(* Logix 5000 Rung export; software revision 16.04 *)

MODULES
   Local : vendor None type None code None
   MVI56E_AFC : vendor None type None code None
END_MODULES

TYPE AFCEComponents :   // High precision gas component analysis (only supported version 2.07.000)
STRUCT
   C1 : REAL;   // Methane
   N2 : REAL;   // Nitrogen
   CO2 : REAL;   // Carbon Dioxide
   C2 : REAL;   // Ethane
   C3 : REAL;   // Propane
   H20 : REAL;   // Water
   H2S : REAL;   // Hydrogen Sulphide
   H2 : REAL;   // Hydrogen
   CO : REAL;   // Carbon Monoxide
   O2 : REAL;   // Oxygen
   IC4 : REAL;   // Iso-butane
   NC4 : REAL;   // Normal Butane
   IC5 : REAL;   // Iso-pentane
   NC5 : REAL;   // Normal-pentane
   C6 : REAL;   // Hexane
   C7 : REAL;   // Heptane
   C8 : REAL;   // Octane
   C9 : REAL;   // Nonane
   C10 : REAL;   // Decane
   He : REAL;   // Helium
   Ar : REAL;   // Argon
   NeoC5 : REAL;   // Not Used
   UxUser1 : REAL;   // Not Used
   UyUser2 : REAL;   // Not Used
   UxUser3 : REAL;   // Not Used
   UyUser4 : REAL;   // Not Used
   UxUser5 : REAL;   // Not Used
   UyUser6 : REAL;   // Not Used
   UxUser7 : REAL;   // Not Used
   UyUser8 : REAL;   // Not Used
   UxUser9 : REAL;   // Not Used
   UyUser10 : REAL;   // Not Used
END_STRUCT
END_TYPE

TYPE AFCEProveProcess :   // Prove process output from processor to the module
STRUCT
   Sequencing : AFCEProveSequencing;   // Prover sequencing
   Temperature : REAL;   // Temperature for Single Probe provers. And Inlet Temperature for Dual Probe Provers.
   OutletTemperature : REAL;   // Outlet Temperature for Provers with Dual Probes.
   SwitchBarTemperature : REAL;   // Switch bar temperature
   Pressure : REAL;   // Pressure for Single Probe provers. And Inlet Pressure for Dual Probe Provers.
   OutletPressure : REAL;   // Outlet Pressure for Provers with Dual Probes.
   ProverDensity : REAL;   // Prover density
END_STRUCT
END_TYPE

TYPE AFCEMeterControl :   // Enable/Disable Meter and Streams
STRUCT
   Meter : AFCEMeterControlMeter;   // Control the Meter
   Stream : AFCEMeterControlStream;   // Control the Meter Streams
   ResetAccumulators : AFCEMeterSignals;   // Resets for meter accumulators
END_STRUCT
END_TYPE

TYPE AFCEMeterDifferentialGasBackPlaneReturn :   // Differential Gas Meter
STRUCT
   StandardDefault : AFCEMeterDifferentialGasStandardDflt;
   StandardRaw : INT[14];
   Extended : AFCEExtended;
END_STRUCT
END_TYPE

TYPE AFCEModbusMasterDataType :   // Modbus master data type
STRUCT
   Bit : BOOL;   // bit type
   Word : BOOL;   // word type (16-bit)
   Long : BOOL;   // long integer (32-bit)
   LongRemote : BOOL;   // long integer (32-bit)
END_STRUCT
END_TYPE

TYPE AFCEProveSequencing :   // AFC prove sequencing tag for phase selection and ball positioning
STRUCT
   Phase : AFCEProvePhaseBitmap;   // AFC phase sequencing
   BallPositionReady : BOOL;   // Ball position: Ready (Udir & Bdir only; fwd leg Bdir)
   BallPositionSealed : BOOL;   // Ball position: Sealed (Udir & Bdir only; fwd leg Bdir)
   BallPositionReadyBwdLeg : BOOL;   // Ball position: Ready bwd leg (Bdir only)
   BallPositionSealedBwdLeg : BOOL;   // Ball position: Sealed bwd leg (Bdir only)
END_STRUCT
END_TYPE

TYPE AFCEUtil :   // Used for internal ladder logic usage. These values must not be changed by user application.
STRUCT
   Flags : AFCEFlag;   // Wallclock update commands
   CycleCounter : INT;   // Reflects current block ID calculated by ladder to be sent to the module
   Buffer : AFCEUtilBuffer;
   Block : AFCEUtilBlock;
END_STRUCT
END_TYPE

TYPE AFCEExtended :
STRUCT
   Trigger : BOOL;
   Data : AFCEExtendedData;
END_STRUCT
END_TYPE

TYPE AFCEModbusGatewayCommand :   // Modbus Gateway Command
STRUCT
   Config : AFCEModbusGatewayConfig;   // Config data to be entered by the user.
   Trigger : BOOL;   // Trigger the Command, when cleared module has responded.
   Data : INT[200];   // Contains modbus data written to the module (write commands)
END_STRUCT
END_TYPE

TYPE AFCEMeterDifferentialGasAlarmControl :   // Differential Gas Process Alarm Control
STRUCT
   DifferentialPressure : AFCEMeterProcessAlarm;   // Differential Pressure Alarms
   FlowRate : AFCEMeterProcessAlarm;   // Flow Rate Alarms
   Temperature : AFCEMeterProcessAlarm;   // Temperature Alarms
   Pressure : AFCEMeterProcessAlarm;   // Pressure Alarms
END_STRUCT
END_TYPE

TYPE AFCEMeterStatusStream :
STRUCT
   Active : INT;   // Current Active Stream
   Enabled : AFCEMeterStatusStreamEnabled;   // Enabled Streams
   Configured : AFCEMeterStatusStreamEnabled;   // Configured Streams
   EnableAlarm : AFCEMeterStatusStreamAlarm;   // Enable Alarms
END_STRUCT
END_TYPE

TYPE AFCEMeterDifferentialGasAlarm :   // Alarm Status and Control
STRUCT
   Control : AFCEMeterDifferentialGasAlarmControl;   // Alarm Control
END_STRUCT
END_TYPE

TYPE AFCEProveRunResults :   // Run results of the prove. Copied from the module to the pocessor
STRUCT
   CountAttempted : INT;   // Run count attempted
   CountCompleted : INT;   // Run count completed
   CountSelected : INT;   // Run count selected
   RunsSelected : INT;   // Bit Mapped Runs selected for calculations from completed runs
   NewMeterFactor : REAL;   // New meter factor
   ChangeInMeterFactor : REAL;   // Change in meter factor
END_STRUCT
END_TYPE

TYPE AFCEModbusMasterSwap :   // Modbus master swap words/ swap bytes
STRUCT
   SwapWords : BOOL;   // Swap words
   SwapBytes : BOOL;   // Swap bytes
END_STRUCT
END_TYPE

TYPE AFCEModbusMaster :   // Modbus Master. Port 3 must be configured as modbus master through AFC Manager to use this feature.
STRUCT
   Enable : BOOL;   // Enable the modbus master funcionality
   CommandIndex : INT;   // Selects which command index will be executed
   Command : AFCEModbusMasterCommand[10];   // Each command contains a specific modbus request to be sent out of the port
END_STRUCT
END_TYPE

TYPE AFCEFlag :   // Flags contains status information updated by ladder and also trigger bits for clock update
STRUCT
   AFCStopped : BOOL;   // Indicates that the module has sent a new input block to be processed by ladder - UPDATED BY LADDER
   AFCInputSequenceNum : INT;   // Meter number (0 -15) associated to blocks 1-16. Used to update "Profile" (meter type and product group.) UPDATED BY LADDER
END_STRUCT
END_TYPE

TYPE AFCEModbusPassThruBitData :   // AFC Modbus Pass-thru Bit Data
STRUCT
   Data : BOOL[2016];   // Contains received data for bit commands
END_STRUCT
END_TYPE

TYPE AFCEUtilBlockInterrupt :
STRUCT
   Now : BOOL;
   ModbusGateway : DINT;
   EnableDisable : BOOL;
   Analysis : DINT;
END_STRUCT
END_TYPE

TYPE AFCEMeterDifferentialGasArchiveFetchT :   // Fetch Archive
STRUCT
   Trigger : BOOL;   // Trigger Archive Fetch
   Age : INT;   // Initial Archive. 0 = Current Archive
   Error : AFCEMeterArchiveFetchError;   // Archive Fetch Error
   Default : AFCEMeterDifferentialGasArchiveDflt;   // Default Archive
   Raw : INT[100];   // Raw Archive
END_STRUCT
END_TYPE

TYPE AFCEFirmwareVersion :
STRUCT
   Major : SINT;   // Major Version number
   Minor : SINT;   // Minor Version number
   Revision : INT;   // Revision
END_STRUCT
END_TYPE

TYPE AFCEModbusGateway :   // Modbus Gateway
STRUCT
   Command : AFCEModbusGatewayCommand[10];   // Modbus gateway commands - contains setup and modbus data
END_STRUCT
END_TYPE

TYPE AFCEMeterCalRequestActionType :
STRUCT
   ZeroShift : BOOL;   // Zero Shift
   SetZero : BOOL;   // Set Zero
   SetSpan : BOOL;   // Set Span
   SetMid1 : BOOL;   // Set Mid 1
   SetMid2 : BOOL;   // Set Mid 2
   SetMid3 : BOOL;   // Set Mid 3
END_STRUCT
END_TYPE

TYPE AFCEUtilBuffer :   // Buffer
STRUCT
   Input : INT[250];   // Input buffer contains the complete block to be copied from the module
   Output : INT[248];   // Output buffer contains data the complete block to be copied to the module
   Process : INT[240];
   ArchiveDay : INT[98];
   ArchiveHour : INT[98];
   Prove : INT[26];
   Analysis : INT[198];
   MeterEnableDisable : INT[4];
   StreamEnable : INT[48];
   StreamDisable : INT[48];
   StreamSelect : INT[32];
   MeterSignals : INT[32];
   Calibration : INT[36];
END_STRUCT
END_TYPE

TYPE AFCEUtilBlock :
STRUCT
   ProcessInput : INT;
   InterruptPending : AFCEUtilBlockInterrupt;
   InterruptComplete : AFCEUtilBlockInterrupt;
   NonInterruptPending : AFCEUtilBlockNonInterrupt;
   NonInterruptComplete : AFCEUtilBlockNonInterrupt;
END_STRUCT
END_TYPE

TYPE AFCEMeterDifferentialGasCalRequestProces :
STRUCT
   DifferentialPressure : BOOL;   // Differential Pressure
   Temperature : BOOL;   // Temperature
   Pressure : BOOL;   // Pressure
END_STRUCT
END_TYPE

TYPE AFCEMeterSignals :   // Meter trigger accumulator and archive resets
STRUCT
   ResetAccumulator1 : BOOL;   // Set to 1 to reset resettable accumulator 1
   ResetAccumulator2 : BOOL;   // Set to 1 to reset resettable accumulator 2
   ResetAccumulator3 : BOOL;   // Set to 1 to reset resettable accumulator 3
   ResetAccumulator4 : BOOL;   // Set to 1 to reset resettable accumulator 4
END_STRUCT
END_TYPE

TYPE AFCEProve :   // Prove
STRUCT
   Process : AFCEProveProcess;   // Process Variables
   Signals : AFCEProveSignals;   // AFC Prove Signals (triggers the proving update)
   Config : AFCEProveConfig;   // AFC Prove Control (configuration settings)
   PulseCounts : AFCEProvePulseCount;   // Pulse counts to be updated at the end of the run/pass
   ConfigInput : AFCEProveInputConfig;   // AFC prover input configuration
   Status : AFCEProveStatus;   // AFC prover status
   ErrorCode : INT;   // Prove error code
   ProveControlsEcho : INT;   // AFC module Echos the state of the Prove Controls
   RequestedMeterEcho : INT;   // AFC module Echos the Meter number requested
   RequestedCurvePointEcho : INT;   // AFC module Echos the requested Curve Point
   RunResults : AFCEProveRunResults;   // Prove and run results
   ProveEnabled : BOOL;   // ON if prove is enabled. This flag is coped from inputbuffer[247]
END_STRUCT
END_TYPE

TYPE AFCEMeterControlStream :
STRUCT
   Selected : SINT;   // Stream to Enable or Disable and/or make active.
   EnableSelected : BOOL;   // Enable the Selected Stream
   DisableSelected : BOOL;   // Disable the Selected Stream
   SetSelectedToActive : BOOL;   // Set Selected to Active Stream
END_STRUCT
END_TYPE

TYPE AFCEProveConfig :   // Controls (configuration settings) associated to the prover
STRUCT
   Enable : AFCEProveConfigEnable;   // Controls at enable
   Accept : AFCEProveConfigAccept;   // Controls at accept
END_STRUCT
END_TYPE

TYPE AFCEWallclock :
STRUCT
   GetAFCTime : BOOL;   // Get current AFC Time
   SetAFCTimeFromPLCTime : BOOL;   // Set AFC time from PLC time. Updates current AFC time
   EnableLocalDateTime : BOOL;   // Enable Local Date Time.
   AFCTime : AFCETime;   // Coordinated Universal Time. Updated by either getting or setting AFC time.
END_STRUCT
END_TYPE

TYPE AFCEMeterDifferentialGasStandardDflt :   // Differential Gas Meter Default Standard Data
STRUCT
   Meter_Alarms : DINT;   // Meter alarms
   NR_Acc_Net_Totalizer : DINT;   // Non-resettable accumulator, net, totalizer (m3)
   NR_Acc_Net_Residue : REAL;   // Non-resettable accumulator, net, residue (m3)
   FlowRate_Net : REAL;   // Flow rate, net (m3/h)
   FlowRate_Gross : REAL;   // Flow rate, gross (m3/h)
   Ifpv : REAL;   // AGA 8, Supercompressibility, Fpv
   Cprime : REAL;   // C-prime
END_STRUCT
END_TYPE

TYPE AFCEMeterCalRequestActionValue :
STRUCT
   ZeroShift : AFCEMeterCalRequestValue;   // Zero Shift
   SetZero : AFCEMeterCalRequestValue;   // Set Zero
   SetSpan : AFCEMeterCalRequestValue;   // Set Span
   SetMid1 : AFCEMeterCalRequestValue;   // Set Mid 1
   SetMid2 : AFCEMeterCalRequestValue;   // Set Mid 2
   SetMid3 : AFCEMeterCalRequestValue;   // Set Mid 3
END_STRUCT
END_TYPE

TYPE AFCEMeterStatus :   // Status
STRUCT
   Meter : AFCEMeterStatusMeter;   // Meter Status
   Stream : AFCEMeterStatusStream;   // Stream Status
END_STRUCT
END_TYPE

TYPE AFCEModbusMasterConfig :   // Modbus master command settings
STRUCT
   Enable : BOOL;   // Set to 1 to enable command (0=disable)
   FunctionType : BOOL;   // Set to 1 to select write command (0=read command)
   RegisterBank : BOOL;   // Set to 1 to select input register (0=holding register)
   DataType : AFCEModbusMasterDataType;   // Select data type format
   SwapOption : AFCEModbusMasterSwap;   // Select byte and word swap (1 = swap, 0 = no swap)
   TypeSwap : INT;   // This value is calculated by ladder logic and must not be modified by user
   SlaveAddress : INT;   // Modbus slave address of remote device
   ModbusAddress : INT;   // Modbus data address on remote slave
   ElementCount : INT;   // Number of data elements (125 words)
   TransactionID : INT;   // Transaction ID. This value is returned to the ReturnedTransaction ID when the response has been received.
END_STRUCT
END_TYPE

TYPE AFCEMeterStatusStreamEnabled :   // Stream Status 1 = Enabled
STRUCT
   Stream1 : BOOL;
   Stream2 : BOOL;
   Stream3 : BOOL;
   Stream4 : BOOL;
   Stream5 : BOOL;
   Stream6 : BOOL;
   Stream7 : BOOL;
   Stream8 : BOOL;
   Stream9 : BOOL;
   Stream10 : BOOL;
   Stream11 : BOOL;
   Stream12 : BOOL;
   Stream13 : BOOL;
   Stream14 : BOOL;
   Stream15 : BOOL;
   Stream16 : BOOL;
END_STRUCT
END_TYPE

TYPE AFCEMeterDifferentialGasArchiveWrite :   // Write Archive
STRUCT
   Daily : BOOL;   // Set to 1 to write daily archive
   Hourly : BOOL;   // Set to 1 to write hourly archive
END_STRUCT
END_TYPE

TYPE AFCEMeterArchiveFetchError :
STRUCT
   ArchiveSelectionInvalid : BOOL;   // Archive File Selection Invalid
   AgeOutsideSize : BOOL;   // Age Outside Configured File Size
   ArchiveNeverWritten : BOOL;   // Age OK but Archive Record Never Written (new or reconfigured meter)
   Reserverd1 : BOOL;
   Reserverd2 : BOOL;
   Reserverd3 : BOOL;
   Reserverd4 : BOOL;
   Reserverd5 : BOOL;
   Reserverd6 : BOOL;
   Reserverd7 : BOOL;
   Reserverd8 : BOOL;
   Reserverd9 : BOOL;
   Reserverd10 : BOOL;
   Reserverd11 : BOOL;
   Reserverd12 : BOOL;
   Reserverd13 : BOOL;
END_STRUCT
END_TYPE

TYPE AFCEMeterDifferentialGasCalRequest :
STRUCT
   ProcessVariable : AFCEMeterDifferentialGasCalRequestProces;   // Process Variable
   ActionType : AFCEMeterCalRequestActionType;   // Action Type
   Value : AFCEMeterCalRequestActionValue;   // Value
   Count : DINT;   // Number of calibration requests
END_STRUCT
END_TYPE

TYPE AFCESiteStatus :   // Site status bits - contains general information about the module - not meter specific
STRUCT
   AFCActive : BOOL;   // AFC active
   ChecksumAlarms : BOOL;   // Checkum alarm active
   Reserved2 : BOOL;
   Reserved3 : BOOL;
   PLCHalted : BOOL;   // PLC in program mode or missing
   CfgChanged : BOOL;   // Configuration changed
   Powerup : BOOL;   // Module powered up
   ColdStart : BOOL;   // Module performed cold start (BBRAM initialized)
   ModbusMasterPending : BOOL;   // Modbus Master Poll Pending
   ModbusMasterComplete : BOOL;   // Modbus Master Poll Complete
   ModbusPassThruPending : BOOL;   // Modbus Pass-thru Input Pending
   CalibrationRequest : BOOL;   // Calibration request from module
   ProverEnabled : BOOL;   // Prover Enabled
   Reserved13 : BOOL;
   Reserved14 : BOOL;
   Reserved15 : BOOL;
END_STRUCT
END_TYPE

TYPE AFCEModuleDef :   // Main user defined data type
STRUCT
   ModbusGateway : AFCEModbusGateway;   // Reads and write data between processor and module modbus table
   ModbusMaster : AFCEModbusMaster;   // Setup modbus master commands to be sent to remote slaves (through Port 3)
   ModbusPassThru : AFCEModbusPassThru;   // Modbus pass-thru data
   SiteStatus : AFCESiteStatus;   // Site status
   MeterAlarms : AFCESiteAlarms;   // Meter Alarms
   Prove : AFCEProve;   // Prover
   Wallclock : AFCEWallclock;   // Set clock and get clock information
   Firmware : AFCEFirmwareVersion;   // Firmware information
   Util : AFCEUtil;   // Used by ladder logic
END_STRUCT
END_TYPE

TYPE AFCEModbusGatewayConfig :   // Modbus Ggateway Configuration
STRUCT
   Enable : BOOL;   // Set to 1 to enable modbus gateway command (0=disable)
   StartRegister : DINT;   // Start modbus address
   RegisterCount : INT;   // Word count (200 max)
   FunctionType : BOOL;   // 0 = read command, 1 = write command
   RegisterType : BOOL;   // 0 = holding register, 1 = input register
   SlaveType : BOOL;   // 0 = primary slave, 1 = virtual slave
END_STRUCT
END_TYPE

TYPE AFCEMeterCalRequestValue :
STRUCT
   Applied : REAL;   // Applied
   Measured : REAL;   // Measured
END_STRUCT
END_TYPE

TYPE AFCEUtilBlockNonInterrupt :
STRUCT
   Now : BOOL;
   ModbusMasterCommand : BOOL;
   ModbusMasterResponse : BOOL;
   Archive : DINT;
   Prover : BOOL;
   PassThru : BOOL;
   Calibration : BOOL;
END_STRUCT
END_TYPE

TYPE AFCEProveConfigAccept :   // Prove controls at accept. If auto-accept is selected must be available at enable
STRUCT
   RequestedInterpolationPoint : INT;   // Requested interpolation point (0 nearest)
   ApplyMFChangeAllStreams : BOOL;   // Apply change in meter factor to all streams
   ApplyMFChangeCurve : BOOL;   // Apply change in meter factor to all curve points
   ApplyNewMF : BOOL;   // CApply new meter factor
END_STRUCT
END_TYPE

TYPE AFCEMeterDifferentialGasProcess :   // Differential Gas Process Variables
STRUCT
   DifferentialPressure : REAL;   // Differential pressure if Primary Input = Differential pressure
   FlowRate : REAL;   // Flow Rate is Primary Input = Flow rate
   Temperature : REAL;   // Temperature
   Pressure : REAL;   // Static pressure
END_STRUCT
END_TYPE

TYPE AFCEProvePhaseBitmap :   // AFC prove phase bitmap
STRUCT
   NotSelected : BOOL;   // Not selected
   Active : BOOL;   // Active, not counting
   CountingPast1stSwitch : BOOL;   // Counting past 1st switch for Udir and forward leg for Bdir)
   Past2ndSwitchFwdLeg : BOOL;   // Past 2nd switch forward leg (bidirectional only)
   Past1stSwithRetLeg : BOOL;   // Past 1st switch return leg (bidirectional only)
   RunComplete : BOOL;   // Run complete. past 2nd switch.
END_STRUCT
END_TYPE

TYPE AFCETime :   // AFC time format used for wallclock update.
STRUCT
   Year : DINT;   // Year
   Month : DINT;   // Month
   Day : DINT;   // Day
   Hour : DINT;   // Hour
   Minute : DINT;   // Minute
   second : DINT;   // Seconds
END_STRUCT
END_TYPE

TYPE AFCEMeterDifferentialGasCal :   // Processor Mediated Calibration
STRUCT
   Request : AFCEMeterDifferentialGasCalRequest;   // Calibration Request from module
   Response : AFCEMeterCalResponse;   // Processor Response
END_STRUCT
END_TYPE

TYPE AFCEMeterDifferentialGasArchive :   // Different Gas Archive
STRUCT
   Write : AFCEMeterDifferentialGasArchiveWrite;
   Fetch : AFCEMeterDifferentialGasArchiveFetch;
END_STRUCT
END_TYPE

TYPE AFCEProveSignals :   // Contains the proving signals that will trigger specific tasks from the module
STRUCT
   EnableProve : BOOL;   // Enables the prove
   AcceptProve : BOOL;   // Accepts the prove
   RejectProve : BOOL;   // Reject the prove
   RunStart : BOOL;   // Starts the run
   RunComplete : BOOL;   // Flags that the run is complete
   RunCancel : BOOL;   // Cancels the run
   RunDelete : BOOL;   // Deletes the run
   PassComplete : BOOL;   // Flag that the pass is complete
   PauseProve : BOOL;   // Pauses the Proving Process
   AbortProve : BOOL;   // Aborts the prove
END_STRUCT
END_TYPE

TYPE AFCEMeterProfile :   // Meter configuration profile
STRUCT
   MeterType : BOOL;   // 0=Differential, 1=Linear
   ProductGroup : BOOL;   // 0=Gas, 1=Liquid
   PrimaryInput : BOOL;   // For differential, 0=Differential Pressure 1=Flow Rate. For Linear, 0=Pulse Count 1=Pulse Frequency
   AOIMismatch : BOOL;   // AOI Meter type does not match module for meter number
END_STRUCT
END_TYPE

TYPE AFCEMeterStatusStreamAlarm :   // Stream Alarms
STRUCT
   StreamOutOfRange : BOOL;   // Requested Stream Number Out of Range
   StreamNotConfigured : BOOL;   // Requested Stream not Configured
   StreamNotEnabled : BOOL;   // Requested Stream not Enabled
   EventLogFull : BOOL;   // Event Log Full, Action not Performed
END_STRUCT
END_TYPE

TYPE AFCEModbusPassThru :   // AFC Modbus Pass-thru
STRUCT
   Enable : BOOL;   // Set to 1 to enable pass-thru functionality (requires AFC Manager setting)
   MessagePresent : BOOL;   // Message present in the response block
   GetMessage : BOOL;   // Get the pass-thru message. When the bit is cleared the message has been transferred to the PLC.
   FunctionBitWrite : BOOL;   // Function bit write
   OverflowError : BOOL;   // Overflow error flag
   ModbusAddress : INT;   // Destination modbus address
   RegisterCount : INT;   // Number of elements associated to command
   ReadDataWord : INT[125];   // Contains received data for word commands
   ReadDataBit : AFCEModbusPassThruBitData;   // Contains received data for bit commands
END_STRUCT
END_TYPE

TYPE AFCEProveInputConfig :   // Prove input block results - prover configuration
STRUCT
   Type : INT;   // Prover type
   Options : INT;   // Prover options
   RunsPerProveTotal : INT;   // Total runs per prove
   RunsPerProveSelected : INT;   // Selected runs per prove
   MaxRunsBeforeAbort : INT;   // Max total runs before abort
   ShortPassesPerRun : INT;   // Short passes per run if bidir = 2 , else 0
END_STRUCT
END_TYPE

TYPE AFCEMeterDifferentialGasArchiveDflt :   // Default Configuration
STRUCT
   ClosingTimestamp : DINT;
   CumulativeActiveStreams : INT;
   CurrentActiveStream : SINT;
   MeterStatus : SINT;
   FlowingPeriod : DINT;
   PeriodDuration : DINT;
   AccumulatorTotalizer : DINT;
   AccumulatorResidue : REAL;
   MeterAlarms : DINT;
   PrimaryInput : REAL;   // Either Differential Pressure or Flow Rate
   Temperature : REAL;
   Pressure : REAL;
   RelativeDensity : REAL;
   ReferenceCompressibility : REAL;
   FlowingCompressibility : REAL;
   Fpv : REAL;
   PressureExtension : REAL;
   CoefficientDischarge : REAL;
   ExpansionFactor : REAL;
   Cprime : REAL;
   MassNRAccumulatorCurrent : REAL;   // Non-resettable
   MassNRAccumulatorOpening : REAL;   // Non-resettable
   EnergyNRAccumulatorCurrent : REAL;   // Non-resettable
   EnergyNRAccumulatorOpening : REAL;   // Non-resettable
   NetNRAccumulatorCurrent : REAL;   // Non-resettable
   NetNRAccumulatorOpening : REAL;   // Non-resettable
   GrossNRAccumulatorCurrent : REAL;   // Non-resettable
   GrossNRAccumulatorOpening : REAL;   // Non-resettable
   MolarFractionComponent01_C1 : REAL;
   MolarFractionComponent02_N2 : REAL;
   MolarFractionComponent03_CO2 : REAL;
   MolarFractionComponent04_C2 : REAL;
   MolarFractionComponent05_C3 : REAL;
   MolarFractionComponent06_H2O : REAL;
   MolarFractionComponent07_H2S : REAL;
   MolarFractionComponent08_H2 : REAL;
   MolarFractionComponent09_CO : REAL;
   MolarFractionComponent10_O2 : REAL;
   MolarFractionComponent11_IC4 : REAL;
   MolarFractionComponent12_NC4 : REAL;
   MolarFractionComponent13_IC5 : REAL;
   MolarFractionComponent14_NC5 : REAL;
   MolarFractionComponent15_C6 : REAL;
   MolarFractionComponent16_C7 : REAL;
   MolarFractionComponent17_C8 : REAL;
   MolarFractionComponent18_C9 : REAL;
   MolarFractionComponent19_C10 : REAL;
   MolarFractionComponent20_He : REAL;
   MolarFractionComponent21_Ar : REAL;
   UserSpecifiedFlowAveraged1 : REAL;
   UserSpecifiedFlowAveraged2 : REAL;
   UserSpecifiedFlowAveraged3 : REAL;
END_STRUCT
END_TYPE

TYPE AFCEProveStatus :   // Status of the prove (returned from the module to the processor)
STRUCT
   ProveAccepted : BOOL;   // Prove was accepted
   MeterFactorApplied : BOOL;   // Meter factor was applied
   MFAppliedToCurve : BOOL;   // Meter factor was applied to all points in the curve
   MFAppliedToStreams : BOOL;   // Meter factor was applied to all streams
   ProveRejectedByCommand : BOOL;   // Prove was rejected by command
   ProveRejectedNoRuns : BOOL;   // Prove was rejected - empty prove (no runs)
   ProveRejectedDivideBy0 : BOOL;   // Prove was rejected - divide by 0
   ProveEnabled : BOOL;   // Prove is enabled
   ProvingRunInProgress : BOOL;   // Proving run is in progress
   ProveRejectedAbort : BOOL;   // Prove rejected: abort
   ProvePaused : BOOL;   // Prove is paused
   RunCancelled : BOOL;   // Run Is cancelled
   RunTimedOut : BOOL;   // Run timed out
END_STRUCT
END_TYPE

TYPE AFCEMeterProcessAlarm :   // Process Alarms
STRUCT
   SetGeneralFail : BOOL;   // Set to indicate General Failure of the Transmitter
   StaleData : BOOL;   // Clear to Indicate new process input data
   SetLowThreshold : BOOL;   // Set to indicate Lower Range Limit Exceeded
   SetHighThreshold : BOOL;   // Set to indicate Upper Range Limit Exceeded
   SetAutoClearStaleData : BOOL;   // Set to automatically clear stale data
END_STRUCT
END_TYPE

TYPE AFCEProveConfigEnable :   // Prove controls at enable
STRUCT
   MeterNumber : INT;   // Meter number requested (1-16)
   AutoAcceptProve : BOOL;   // Auto-accept the prove
   AutoContinueProve : BOOL;   // Auto-continue the prove
END_STRUCT
END_TYPE

TYPE AFCEMeterAnalysis :   // Meter analysis components. Allows the processor to update molar analysis for low precision and high precision streams.
STRUCT
   Trigger : BOOL;   // Set to 1 to Send Updated Component Data to the Module
   Stream : INT;   // Stream for Analysis. Select 0 for current active stream.
   Error : AFCEMeterAnalysisError;   // Analysis Error
   Components : AFCEComponents;   // High precision gas components (floating point per component). Only supported for firmware version 2.07.000 or later
END_STRUCT
END_TYPE

TYPE AFCEMeterStatusMeter :   // Meter Status
STRUCT
   Enabled : BOOL;   // Meter Enable Status, 1=enabled
   EnableAlarm : BOOL;   // If set either: 1. The meter is not configured. 2. The event log is full, the action was not performed.
END_STRUCT
END_TYPE

TYPE AFCEMeterControlMeter :   // Enable and Disable Meter
STRUCT
   Enable : BOOL;   // Enable the Meter
   Disable : BOOL;   // Disable the Meter
END_STRUCT
END_TYPE

TYPE AFCEMeterDifferentialGas :   // Differential Gas Meter
STRUCT
   Control : AFCEMeterControl;   // Meter Control
   Status : AFCEMeterStatus;   // Meter Status
   ProcessVariables : AFCEMeterDifferentialGasProcess;   // Input process variables to be transferred to the module
   Analysis : AFCEMeterAnalysis;   // Molar Analysis data to be transferred to the module (only for gas products with online gas chromatograph applications)
   Alarm : AFCEMeterDifferentialGasAlarm;   // Meter Alarm status and control
   Archive : AFCEMeterDifferentialGasArchive;   // Archive
   Profile : AFCEMeterProfile;   // Module profile (meter type/product group) transfered from the module
   Calibration : AFCEMeterDifferentialGasCal;   // Calibration
   BackPlaneReturn : AFCEMeterDifferentialGasBackPlaneReturn;
END_STRUCT
END_TYPE

TYPE AFCEModbusMasterCommand :   // Modbus Master Command
STRUCT
   Config : AFCEModbusMasterConfig;   // Modbus Master Configuration
   ErrorCode : INT;   // Error Code associated to Modbus Master Command
   Pending : BOOL;   // Pending Modbus Master Command - waiting for Modbus Response
   ReturnedTransactionID : DINT;   // Changes to Config.TransactionID value when response has returned.
   Data : INT[100];   // Read or Write Data
END_STRUCT
END_TYPE

TYPE AFCEMeterDifferentialGasArchiveFetch :
STRUCT
   Daily : AFCEMeterDifferentialGasArchiveFetchT;
   Hourly : AFCEMeterDifferentialGasArchiveFetchT;
END_STRUCT
END_TYPE

TYPE AFCEProvePulseCount :   // Values to be supplied at the end of the pass/run
STRUCT
   Meter : DINT;   // Meter pulse count
   MasterMeter : DINT;   // Master meter pulse count
END_STRUCT
END_TYPE

TYPE AFCEMeterCalResponse :
STRUCT
   Trigger : BOOL;   // Send Error Code and Values to module to be recorded
   ErrorCode : SINT;   // Error Code to send. 0-4 allowed. 0=No error. 1-4=User defined.
   Value : AFCEMeterCalRequestValue;   // Value to Send
   Count : DINT;   // Number of calibration responses
END_STRUCT
END_TYPE

TYPE AFCEExtendedData :
STRUCT
   Raw : INT[64];
END_STRUCT
END_TYPE

TYPE AFCESiteAlarms :   // Indicates if a meter has any alarms
STRUCT
   Meter1 : BOOL;   // Meter in alarm
   Meter2 : BOOL;   // Meter in alarm
   Meter3 : BOOL;   // Meter in alarm
   Meter4 : BOOL;   // Meter in alarm
   Meter5 : BOOL;   // Meter in alarm
   Meter6 : BOOL;   // Meter in alarm
   Meter7 : BOOL;   // Meter in alarm
   Meter8 : BOOL;   // Meter in alarm
   Meter9 : BOOL;   // Meter in alarm
   Meter10 : BOOL;   // Meter in alarm
   Meter11 : BOOL;   // Meter in alarm
   Meter12 : BOOL;   // Meter in alarm
   Meter13 : BOOL;   // Meter in alarm
   Meter14 : BOOL;   // Meter in alarm
   Meter15 : BOOL;   // Meter in alarm
   Meter16 : BOOL;   // Meter in alarm
END_STRUCT
END_TYPE

TYPE AFCEMeterAnalysisError :
STRUCT
   StreamOutOfRange : BOOL;   // Requested Stream Number Out of Range
   StreamNotConfigured : BOOL;   // Requested Stream Not Configured
END_STRUCT
END_TYPE

ADD_ON_INSTRUCTION AOI56EAFCMeterDifferentialGas   (* revision 1.8, vendor ProSoft Technology Inc., ExecutePrescan *)
// Add-On instruction for the MVI56E-AFC.
// Differential Gas Meter
// Revision note:
// Corrected/Reverted ProcessInputBlockID Tag Data Type from INT to DINT.
// Help:
// Compatible with version 4.03 of MVI56E-AFC firmware or higher.
// v1.2: Remove Calculation Results. Add Backplane Return. Add Stale Data
// v1.3: Added Flow Rate Process Input and Flow Rate Alarm Controller Tags for Flow Rate Devices (and not just for Differential Pressure)
// v1.4: Addition of default process input backplane return data mapping.
// v1.5: Made correlation changes between the Module Archive Default UDTs and the AOI Archive Default UDTs.
// v1.6: Made changes to the Flow Rate Primary Input Block ID Insertion in Rung 8 (Removed +1),
// Modified ProcessInputBlockID Tag Data Type from DINT to INT. and modified ModbusGatewayConfig UDT StartRegister Tag Data Type from INT to DINT.
// v1.7:  Updated Tags names AFCMeterXXYYYYYY.BackPlaneReturn.ProcessInputs to AFCMeterXXYYYYYY.BackPlaneReturn.Standard and AFCMeterXXYYYYYY.BackPlaneReturn.ComponentAnalysis
//  to AFCMeterXXYYYYYY.BackPlaneReturn.Extended
// v1.8:  Corrected/Reverted ProcessInputBlockID Tag Data Type from INT to DINT.
VAR_IN_OUT
   ConnectionInput : INT[250]; {required}
   AFC : AFCEModuleDef; {required}
   AFCMeter : AFCEMeterDifferentialGas; {required}
END_VAR
VAR_INPUT
   MeterNumber : SINT; {required}   // Meter Number Set to a number between 1 and 16
END_VAR
VAR
   TimestampBuffer : DINT;
   StreamSelectedShift : DINT;
   StreamSelectBuffer : INT;
   EnabledStatusBuffer : INT;
   StreamSelectBlockID : DINT;
   StreamNumberShift : DINT;
   StreamErrorBuffer : DINT;
   StreamEnableBlockID : DINT;
   StreamEnableBitPosition : DINT;
   StreamDisableBlockID : DINT;
   ProfileBuffer : SINT[2];
   ProcessInputBlockID : DINT;
   CalibrationHandleBuffer : INT;
   AnalysisGroupBitPosition : INT;
   ProcessAlarmShifter : DINT;
   ProcessAlarmBuffer : DINT;
   MeterSignaltBlockID : DINT;
   MeterNumberShift : DINT;
   MeterNumberBitPostition : DINT;
   Inputbuffer : INT[250];
   CurrentHourlyAgeONS : BOOL;
   CurrentHourlyAge : DINT;
   CurrentDailyAgeONS : BOOL;
   CurrentDailyAge : DINT;
   ClearMeterSignal : BOOL;   // Repeat the meter signal block with cleared signal bits. This allows repeat triggering of a signal.
   CalibrationMeterNumberBuffer : DINT;
   CalibrationMediationPending : BOOL;
   CalibrationInputScalingIndex : DINT;
   AnalysisErrorBuffer : INT;
   ArchiveStream : DINT;
   ArchiveMeterStatusRaw : DINT;
   ArchiveMeterStatusActiveStream : DINT;
   ArchiveHourlyRawSize : DINT;
   ArchiveHourlyOffset : DINT;
   ArchiveHourlyDefaultSize : DINT;
   ArchiveDailyRawSize : DINT;
   ArchiveDailyOffset : DINT;
   ArchiveDailyDefaultSize : DINT;
   ArchiveCompleteBitCheck : DINT;
   ArchiveBlockID : DINT;
   AnalysisGroupShift : DINT;
   AnalysisCompleteBitCheck : DINT;
   AnalysisBufferOffset : DINT;
   AnalysisBlockID : DINT;
   AFCStopped : BOOL;
   AFCInputDataAvailable : BOOL;
END_VAR

ROUTINE Logic   (* ladder *)
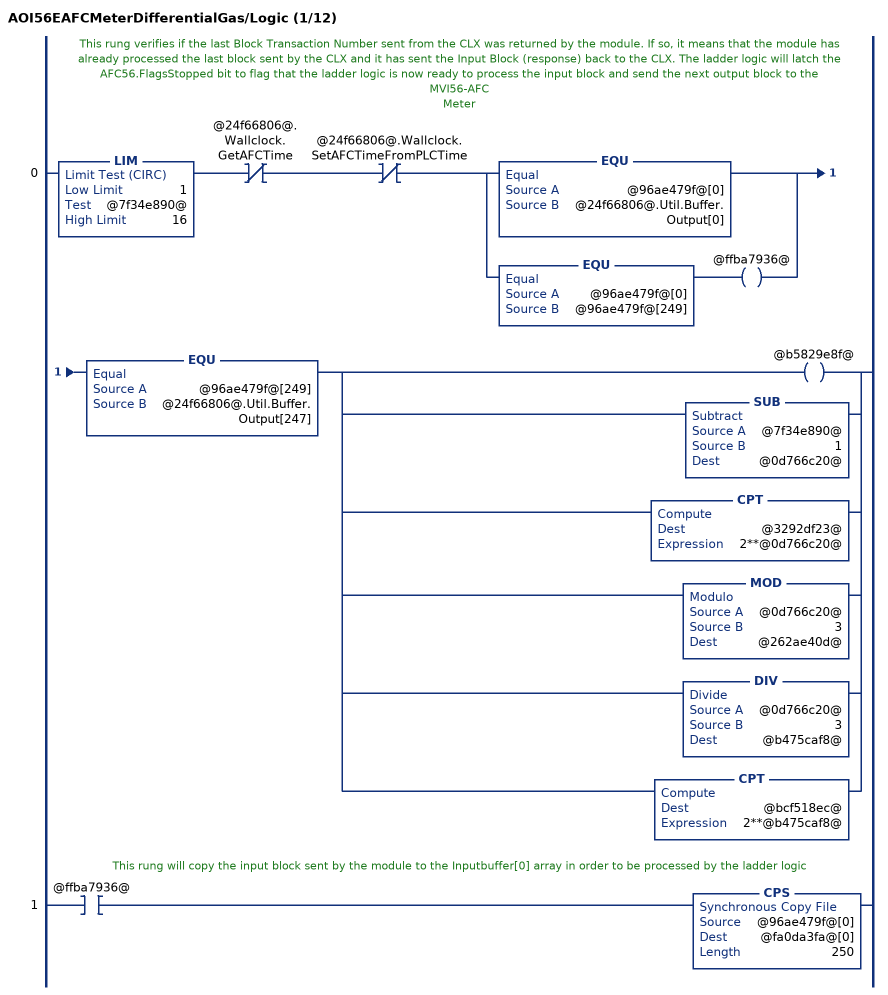
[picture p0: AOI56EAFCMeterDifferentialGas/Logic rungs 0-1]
   // This rung verifies if the last Block Transaction Number sent from the CLX was returned by the module. If so, it means that the module has already processed the last block sent by the CLX and it has sent the Input Block (response) back to the CLX. The ladder logic will latch the AFC56.FlagsStopped bit to flag that the ladder logic is now ready to process the input block and send the next output block to the MVI56-AFC
   // Meter
   0: LIM(1,@7f34e890@,16)XIO(@24f66806@.Wallclock.GetAFCTime)XIO(@24f66806@.Wallclock.SetAFCTimeFromPLCTime)[EQU(@96ae479f@[0],@24f66806@.Util.Buffer.Output[0]) ,EQU(@96ae479f@[0],@96ae479f@[249]) OTE(@ffba7936@) ]EQU(@96ae479f@[249],@24f66806@.Util.Buffer.Output[247])[OTE(@b5829e8f@) ,SUB(@7f34e890@,1,@0d766c20@) ,CPT(@3292df23@,2**@0d766c20@) ,MOD(@0d766c20@,3,@262ae40d@) ,DIV(@0d766c20@,3,@b475caf8@) ,CPT(@bcf518ec@,2**@b475caf8@) ];
   // This rung will copy the input block sent by the module to the Inputbuffer[0] array in order to be processed by the ladder logic
   1: XIC(@ffba7936@)CPS(@96ae479f@[0],@fa0da3fa@[0],250);
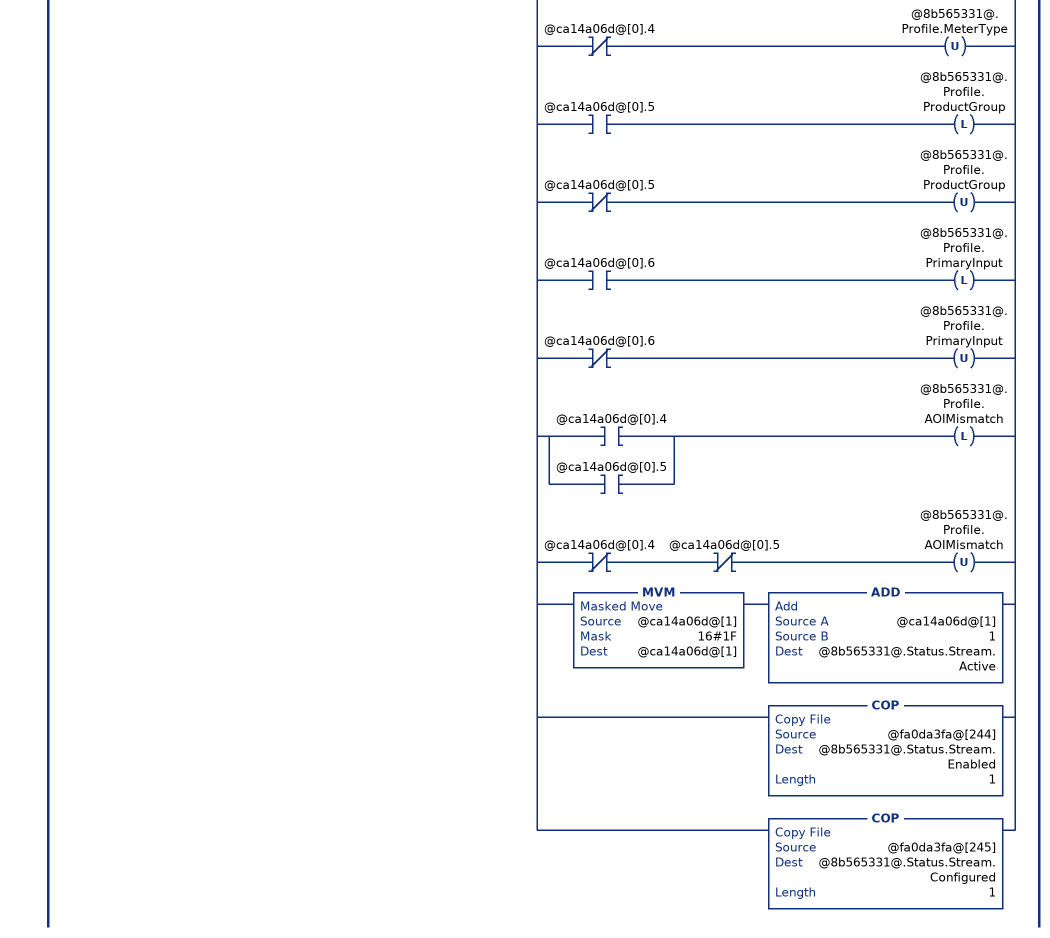
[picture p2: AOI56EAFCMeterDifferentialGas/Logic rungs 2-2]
   // Read process input backplane return and
   // meter profile (when block ID matches meter number).
   2: XIC(@ffba7936@)LIM(1,@fa0da3fa@[0],16)[COP(@fa0da3fa@[3+@0d766c20@*15],@8b565331@.BackPlaneReturn.StandardRaw[0],14) ,COP(@8b565331@.BackPlaneReturn.StandardRaw[0],@8b565331@.BackPlaneReturn.StandardDefault,1) ,COP(@fa0da3fa@[247],@24f66806@.SiteStatus,1) ,COP(@fa0da3fa@[248],@24f66806@.MeterAlarms,1) ,EQU(@fa0da3fa@[0],@7f34e890@) [COP(@fa0da3fa@[243],@ca14a06d@[0],2) ,[XIC(@ca14a06d@[0].0) OTL(@8b565331@.Status.Meter.EnableAlarm) ,XIO(@ca14a06d@[0].0) OTU(@8b565331@.Status.Meter.EnableAlarm) ] ,[XIC(@ca14a06d@[0].1) OTL(@8b565331@.Status.Meter.Enabled) ,XIO(@ca14a06d@[0].1) OTU(@8b565331@.Status.Meter.Enabled) ] ,[[XIC(@ca14a06d@[0].4) OTL(@8b565331@.Profile.MeterType) ,XIO(@ca14a06d@[0].4) OTU(@8b565331@.Profile.MeterType) ] ,[XIC(@ca14a06d@[0].5) OTL(@8b565331@.Profile.ProductGroup) ,XIO(@ca14a06d@[0].5) OTU(@8b565331@.Profile.ProductGroup) ] ,[XIC(@ca14a06d@[0].6) OTL(@8b565331@.Profile.PrimaryInput) ,XIO(@ca14a06d@[0].6) OTU(@8b565331@.Profile.PrimaryInput) ] ] ,[[XIC(@ca14a06d@[0].4) ,XIC(@ca14a06d@[0].5) ] OTL(@8b565331@.Profile.AOIMismatch) ,XIO(@ca14a06d@[0].4) XIO(@ca14a06d@[0].5) OTU(@8b565331@.Profile.AOIMismatch) ] ,MVM(@ca14a06d@[1],16#1F,@ca14a06d@[1]) ADD(@ca14a06d@[1],1,@8b565331@.Status.Stream.Active) ,COP(@fa0da3fa@[244],@8b565331@.Status.Stream.Enabled,1) ,COP(@fa0da3fa@[245],@8b565331@.Status.Stream.Configured,1) ] ];
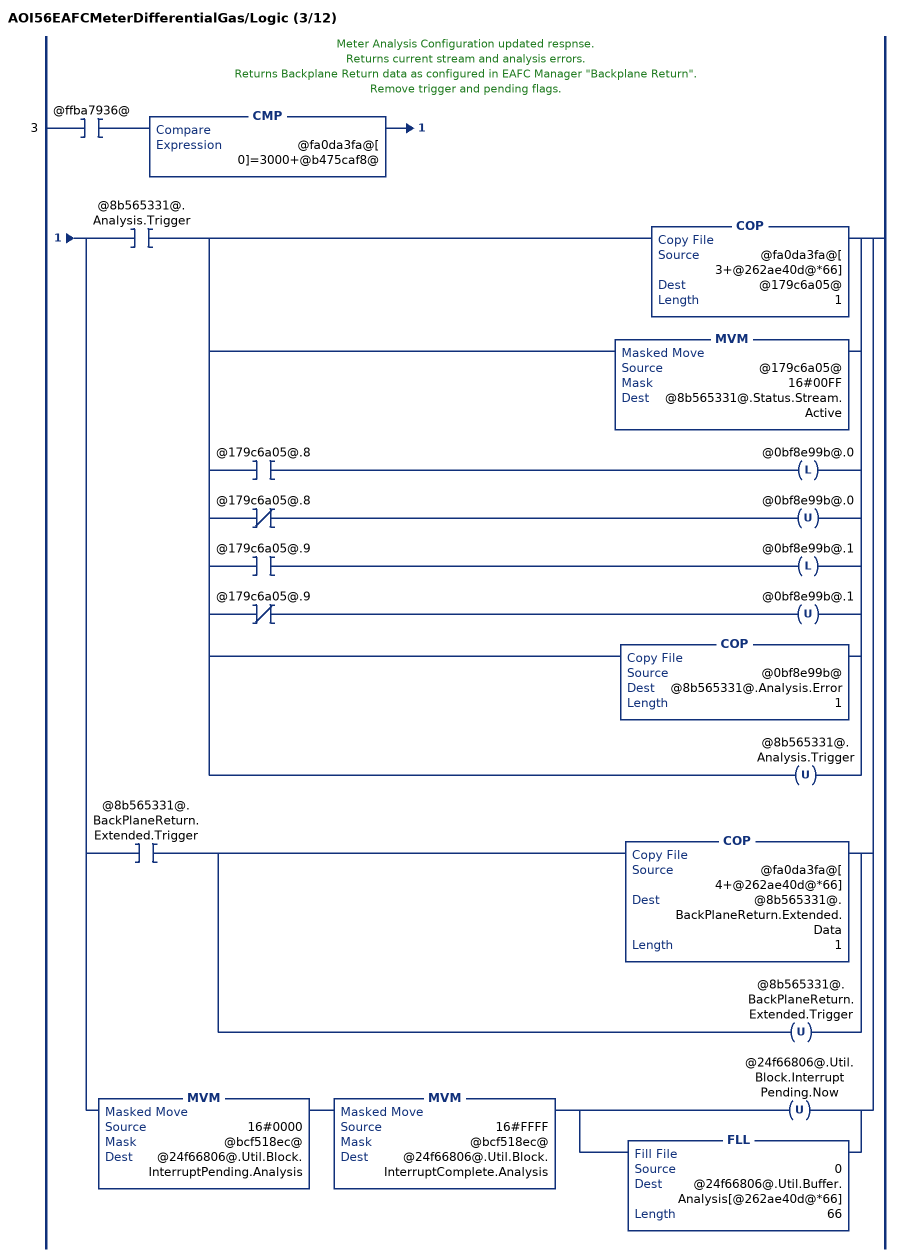
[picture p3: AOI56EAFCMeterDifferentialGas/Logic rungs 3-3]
   // Meter Analysis Configuration updated respnse.
   // Returns current stream and analysis errors.
   // Returns Backplane Return data as configured in EAFC Manager "Backplane Return".
   // Remove trigger and pending flags.
   3: XIC(@ffba7936@)CMP(@fa0da3fa@[0]=3000+@b475caf8@)[XIC(@8b565331@.Analysis.Trigger) [COP(@fa0da3fa@[3+@262ae40d@*66],@179c6a05@,1) ,MVM(@179c6a05@,16#00FF,@8b565331@.Status.Stream.Active) ,[XIC(@179c6a05@.8) OTL(@0bf8e99b@.0) ,XIO(@179c6a05@.8) OTU(@0bf8e99b@.0) ] ,[XIC(@179c6a05@.9) OTL(@0bf8e99b@.1) ,XIO(@179c6a05@.9) OTU(@0bf8e99b@.1) ] ,COP(@0bf8e99b@,@8b565331@.Analysis.Error,1) ,OTU(@8b565331@.Analysis.Trigger) ] ,XIC(@8b565331@.BackPlaneReturn.Extended.Trigger) [COP(@fa0da3fa@[4+@262ae40d@*66],@8b565331@.BackPlaneReturn.Extended.Data,1) ,OTU(@8b565331@.BackPlaneReturn.Extended.Trigger) ] ,MVM(16#0000,@bcf518ec@,@24f66806@.Util.Block.InterruptPending.Analysis) MVM(16#FFFF,@bcf518ec@,@24f66806@.Util.Block.InterruptComplete.Analysis) [OTU(@24f66806@.Util.Block.InterruptPending.Now) ,FLL(0,@24f66806@.Util.Buffer.Analysis[@262ae40d@*66],66) ] ];
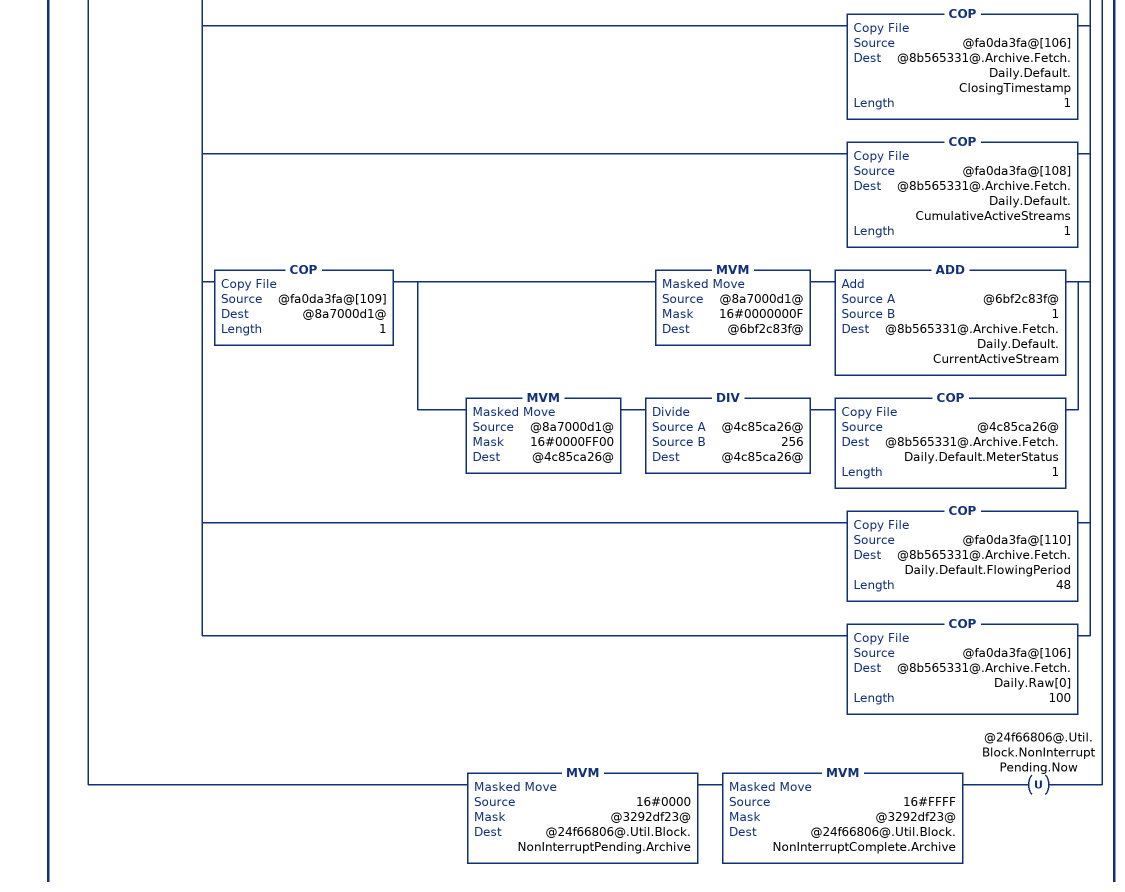
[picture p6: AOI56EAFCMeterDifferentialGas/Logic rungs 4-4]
   // Archive Fetch to default and raw UDT's.
   // Get archive alarms.
   // Remove trigger and pending flags.
   4: XIC(@ffba7936@)CMP(@fa0da3fa@[0]=6000+@0d766c20@)[XIC(@8b565331@.Archive.Fetch.Hourly.Trigger) [OTU(@8b565331@.Archive.Fetch.Hourly.Trigger) ,[[XIC(@fa0da3fa@[3].0) OTL(@8b565331@.Archive.Fetch.Hourly.Error.ArchiveSelectionInvalid) ,XIO(@fa0da3fa@[3].0) OTU(@8b565331@.Archive.Fetch.Hourly.Error.ArchiveSelectionInvalid) ] ,[XIC(@fa0da3fa@[3].1) OTL(@8b565331@.Archive.Fetch.Hourly.Error.AgeOutsideSize) ,XIO(@fa0da3fa@[3].1) OTU(@8b565331@.Archive.Fetch.Hourly.Error.AgeOutsideSize) ] ,[XIC(@fa0da3fa@[3].2) OTL(@8b565331@.Archive.Fetch.Hourly.Error.ArchiveNeverWritten) ,XIO(@fa0da3fa@[3].2) OTU(@8b565331@.Archive.Fetch.Hourly.Error.ArchiveNeverWritten) ] ] ,COP(@fa0da3fa@[4],@8b565331@.Archive.Fetch.Hourly.Default.ClosingTimestamp,1) ,COP(@fa0da3fa@[6],@8b565331@.Archive.Fetch.Hourly.Default.CumulativeActiveStreams,1) ,COP(@fa0da3fa@[7],@8a7000d1@,1) [MVM(@8a7000d1@,16#0000000F,@6bf2c83f@) ADD(@6bf2c83f@,1,@8b565331@.Archive.Fetch.Hourly.Default.CurrentActiveStream) ,MVM(@8a7000d1@,16#0000FF00,@4c85ca26@) DIV(@4c85ca26@,256,@4c85ca26@) COP(@4c85ca26@,@8b565331@.Archive.Fetch.Hourly.Default.MeterStatus,1) ] ,COP(@fa0da3fa@[8],@8b565331@.Archive.Fetch.Hourly.Default.FlowingPeriod,48) ,COP(@fa0da3fa@[4],@8b565331@.Archive.Fetch.Hourly.Raw[0],100) ] ,XIC(@8b565331@.Archive.Fetch.Daily.Trigger) [OTU(@8b565331@.Archive.Fetch.Daily.Trigger) ,[[XIC(@fa0da3fa@[105].0) OTL(@8b565331@.Archive.Fetch.Daily.Error.ArchiveSelectionInvalid) ,XIO(@fa0da3fa@[105].0) OTU(@8b565331@.Archive.Fetch.Daily.Error.ArchiveSelectionInvalid) ] ,[XIC(@fa0da3fa@[105].1) OTL(@8b565331@.Archive.Fetch.Daily.Error.AgeOutsideSize) ,XIO(@fa0da3fa@[105].1) OTU(@8b565331@.Archive.Fetch.Daily.Error.AgeOutsideSize) ] ,[XIC(@fa0da3fa@[105].2) OTL(@8b565331@.Archive.Fetch.Daily.Error.ArchiveNeverWritten) ,XIO(@fa0da3fa@[105].2) OTU(@8b565331@.Archive.Fetch.Daily.Error.ArchiveNeverWritten) ] ] ,COP(@fa0da3fa@[106],@8b565331@.Archive.Fetch.Daily.Default.ClosingTimestamp,1) ,COP(@fa0da3fa@[108],@8b565331@.Archive.Fetch.Daily.Default.CumulativeActiveStreams,1) ,COP(@fa0da3fa@[109],@8a7000d1@,1) [MVM(@8a7000d1@,16#0000000F,@6bf2c83f@) ADD(@6bf2c83f@,1,@8b565331@.Archive.Fetch.Daily.Default.CurrentActiveStream) ,MVM(@8a7000d1@,16#0000FF00,@4c85ca26@) DIV(@4c85ca26@,256,@4c85ca26@) COP(@4c85ca26@,@8b565331@.Archive.Fetch.Daily.Default.MeterStatus,1) ] ,COP(@fa0da3fa@[110],@8b565331@.Archive.Fetch.Daily.Default.FlowingPeriod,48) ,COP(@fa0da3fa@[106],@8b565331@.Archive.Fetch.Daily.Raw[0],100) ] ,MVM(16#0000,@3292df23@,@24f66806@.Util.Block.NonInterruptPending.Archive) MVM(16#FFFF,@3292df23@,@24f66806@.Util.Block.NonInterruptComplete.Archive) OTU(@24f66806@.Util.Block.NonInterruptPending.Now) ];
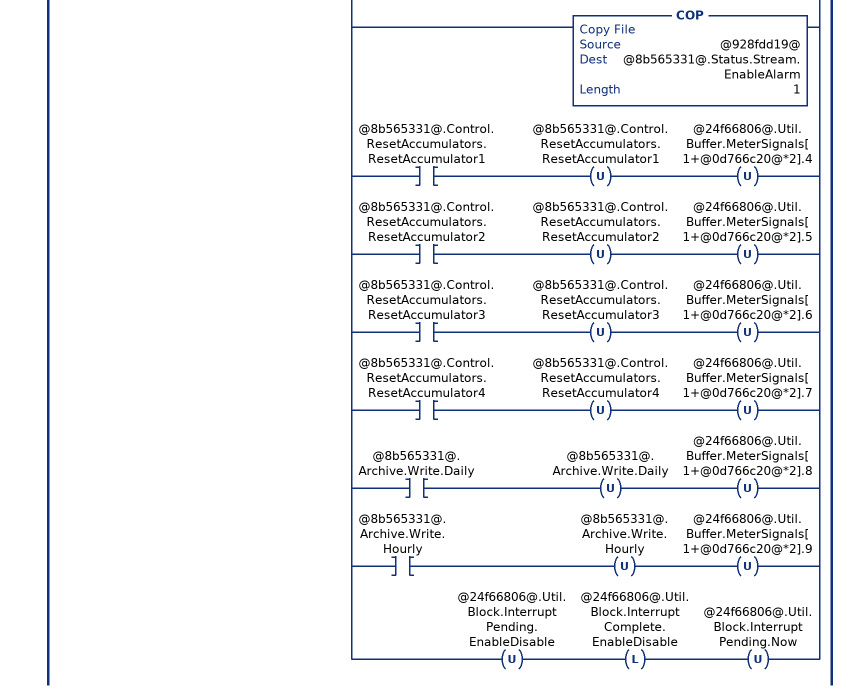
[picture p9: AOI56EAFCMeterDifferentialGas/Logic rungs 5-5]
   // Meter status and stream status.
   // Remove trigger and pending flags.
   5: XIC(@ffba7936@)EQU(@fa0da3fa@[0],7000)[[MVM(@fa0da3fa@[3],@3292df23@,@5b497894@) ,[NEQ(@5b497894@,0) OTL(@8b565331@.Status.Meter.Enabled) ,EQU(@5b497894@,0) OTU(@8b565331@.Status.Meter.Enabled) ] ,OTU(@8b565331@.Control.Meter.Enable) MVM(16#0000,@3292df23@,@24f66806@.Util.Buffer.MeterEnableDisable[1]) ,OTU(@8b565331@.Control.Meter.Disable) MVM(16#0000,@3292df23@,@24f66806@.Util.Buffer.MeterEnableDisable[3]) ] ,[XIC(@8b565331@.Control.Stream.EnableSelected) [COP(@fa0da3fa@[7+@0d766c20@*3],@8b565331@.Status.Stream.Enabled,1) ,COP(@fa0da3fa@[8+@0d766c20@*3],@8b565331@.Status.Stream.Configured,1) ,OTU(@8b565331@.Control.Stream.EnableSelected) OTU(@8b565331@.Control.Stream.DisableSelected) ] ,XIC(@8b565331@.Control.Stream.DisableSelected) [COP(@fa0da3fa@[55+@0d766c20@*3],@8b565331@.Status.Stream.Enabled,1) ,COP(@fa0da3fa@[56+@0d766c20@*3],@8b565331@.Status.Stream.Configured,1) ,OTU(@8b565331@.Control.Stream.EnableSelected) OTU(@8b565331@.Control.Stream.DisableSelected) ] ] ,[OTU(@8b565331@.Control.Stream.SetSelectedToActive) ,COP(@fa0da3fa@[103+@0d766c20@*2],@179c6a05@,1) ,[XIC(@179c6a05@.8) OTL(@928fdd19@.0) ,XIO(@179c6a05@.8) OTU(@928fdd19@.0) ] ,[XIC(@179c6a05@.9) OTL(@928fdd19@.1) ,XIO(@179c6a05@.9) OTU(@928fdd19@.1) ] ,[XIC(@179c6a05@.10) OTL(@928fdd19@.2) ,XIO(@179c6a05@.10) OTU(@928fdd19@.2) ] ,[XIC(@179c6a05@.11) OTL(@928fdd19@.3) ,XIO(@179c6a05@.11) OTU(@928fdd19@.3) ] ,MVM(@179c6a05@,16#000F,@a9249fea@) ADD(@a9249fea@,1,@8b565331@.Status.Stream.Active) ,COP(@928fdd19@,@8b565331@.Status.Stream.EnableAlarm,1) ] ,[XIC(@8b565331@.Control.ResetAccumulators.ResetAccumulator1) OTU(@8b565331@.Control.ResetAccumulators.ResetAccumulator1) OTU(@24f66806@.Util.Buffer.MeterSignals[1+@0d766c20@*2].4) ,XIC(@8b565331@.Control.ResetAccumulators.ResetAccumulator2) OTU(@8b565331@.Control.ResetAccumulators.ResetAccumulator2) OTU(@24f66806@.Util.Buffer.MeterSignals[1+@0d766c20@*2].5) ,XIC(@8b565331@.Control.ResetAccumulators.ResetAccumulator3) OTU(@8b565331@.Control.ResetAccumulators.ResetAccumulator3) OTU(@24f66806@.Util.Buffer.MeterSignals[1+@0d766c20@*2].6) ,XIC(@8b565331@.Control.ResetAccumulators.ResetAccumulator4) OTU(@8b565331@.Control.ResetAccumulators.ResetAccumulator4) OTU(@24f66806@.Util.Buffer.MeterSignals[1+@0d766c20@*2].7) ,XIC(@8b565331@.Archive.Write.Daily) OTU(@8b565331@.Archive.Write.Daily) OTU(@24f66806@.Util.Buffer.MeterSignals[1+@0d766c20@*2].8) ,XIC(@8b565331@.Archive.Write.Hourly) OTU(@8b565331@.Archive.Write.Hourly) OTU(@24f66806@.Util.Buffer.MeterSignals[1+@0d766c20@*2].9) ] ,OTU(@24f66806@.Util.Block.InterruptPending.EnableDisable) OTL(@24f66806@.Util.Block.InterruptComplete.EnableDisable) OTU(@24f66806@.Util.Block.InterruptPending.Now) ];
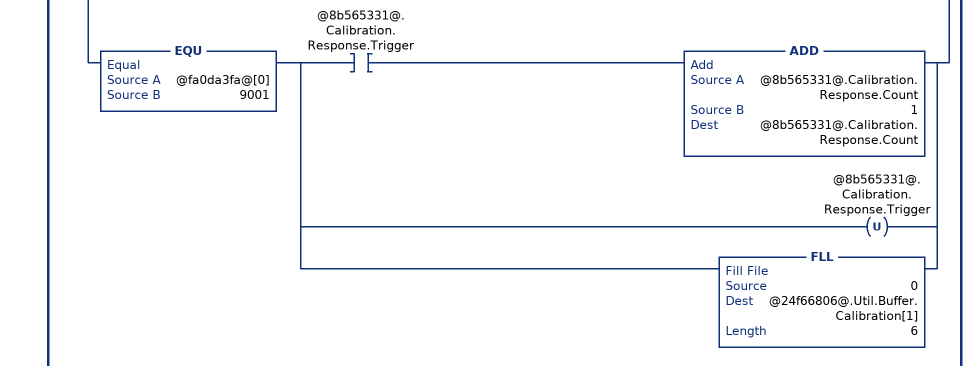
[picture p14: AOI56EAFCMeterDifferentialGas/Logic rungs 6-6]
   // Meter transmitter calibration.
   6: XIC(@ffba7936@)[EQU(@fa0da3fa@[0],9000) ,EQU(@fa0da3fa@[0],9001) ][MVM(@fa0da3fa@[3],16#0F00,@27a67968@) ,DIV(@27a67968@,16#100,@27a67968@) ]EQU(@27a67968@,@0d766c20@)XIO(@fa0da3fa@[3].14)[EQU(@fa0da3fa@[0],9000) [XIO(@3834a44b@) ADD(@8b565331@.Calibration.Request.Count,1,@8b565331@.Calibration.Request.Count) ,OTL(@3834a44b@) [COP(@fa0da3fa@[3],@0762a03d@,1) ,MVM(@0762a03d@,16#000F,@264aad82@) ] ,[EQU(@264aad82@,0) [OTL(@8b565331@.Calibration.Request.ProcessVariable.DifferentialPressure) ,OTU(@8b565331@.Calibration.Request.ProcessVariable.Temperature) ,OTU(@8b565331@.Calibration.Request.ProcessVariable.Pressure) ] ,EQU(@264aad82@,1) [OTL(@8b565331@.Calibration.Request.ProcessVariable.Temperature) ,OTU(@8b565331@.Calibration.Request.ProcessVariable.DifferentialPressure) ,OTU(@8b565331@.Calibration.Request.ProcessVariable.Pressure) ] ,EQU(@264aad82@,2) [OTL(@8b565331@.Calibration.Request.ProcessVariable.Pressure) ,OTU(@8b565331@.Calibration.Request.ProcessVariable.DifferentialPressure) ,OTU(@8b565331@.Calibration.Request.ProcessVariable.Temperature) ] ] ,[[XIC(@fa0da3fa@[5].2) [OTL(@8b565331@.Calibration.Request.ActionType.ZeroShift) ,COP(@fa0da3fa@[6],@8b565331@.Calibration.Request.Value.ZeroShift.Applied,2) ] ,XIO(@fa0da3fa@[5].2) [OTU(@8b565331@.Calibration.Request.ActionType.ZeroShift) ,FLL(0,@8b565331@.Calibration.Request.Value.ZeroShift.Applied,2) ] ] ,[XIC(@fa0da3fa@[5].3) [OTL(@8b565331@.Calibration.Request.ActionType.SetZero) ,COP(@fa0da3fa@[10],@8b565331@.Calibration.Request.Value.SetZero.Applied,2) ] ,XIO(@fa0da3fa@[5].3) [OTU(@8b565331@.Calibration.Request.ActionType.SetZero) ,FLL(0,@8b565331@.Calibration.Request.Value.SetZero.Applied,2) ] ] ,[XIC(@fa0da3fa@[5].4) [OTL(@8b565331@.Calibration.Request.ActionType.SetSpan) ,COP(@fa0da3fa@[14],@8b565331@.Calibration.Request.Value.SetSpan.Applied,2) ] ,XIO(@fa0da3fa@[5].4) [OTU(@8b565331@.Calibration.Request.ActionType.SetSpan) ,FLL(0,@8b565331@.Calibration.Request.Value.SetSpan.Applied,2) ] ] ,[XIC(@fa0da3fa@[5].5) [OTL(@8b565331@.Calibration.Request.ActionType.SetMid1) ,COP(@fa0da3fa@[18],@8b565331@.Calibration.Request.Value.SetMid1.Applied,2) ] ,XIO(@fa0da3fa@[5].5) [OTU(@8b565331@.Calibration.Request.ActionType.SetMid1) ,FLL(0,@8b565331@.Calibration.Request.Value.SetMid1.Applied,2) ] ] ,[XIC(@fa0da3fa@[5].6) [OTL(@8b565331@.Calibration.Request.ActionType.SetMid2) ,COP(@fa0da3fa@[22],@8b565331@.Calibration.Request.Value.SetMid2.Applied,2) ] ,XIO(@fa0da3fa@[5].6) [OTU(@8b565331@.Calibration.Request.ActionType.SetMid2) ,FLL(0,@8b565331@.Calibration.Request.Value.SetMid2.Applied,2) ] ] ,[XIC(@fa0da3fa@[5].7) [OTL(@8b565331@.Calibration.Request.ActionType.SetMid3) ,COP(@fa0da3fa@[26],@8b565331@.Calibration.Request.Value.SetMid3.Applied,2) ] ,XIO(@fa0da3fa@[5].7) [OTU(@8b565331@.Calibration.Request.ActionType.SetMid3) ,FLL(0,@8b565331@.Calibration.Request.Value.SetMid3.Applied,2) ] ] ] ] ,EQU(@fa0da3fa@[0],9001) [XIC(@8b565331@.Calibration.Response.Trigger) ADD(@8b565331@.Calibration.Response.Count,1,@8b565331@.Calibration.Response.Count) ,OTU(@8b565331@.Calibration.Response.Trigger) ,FLL(0,@24f66806@.Util.Buffer.Calibration[1],6) ] ];
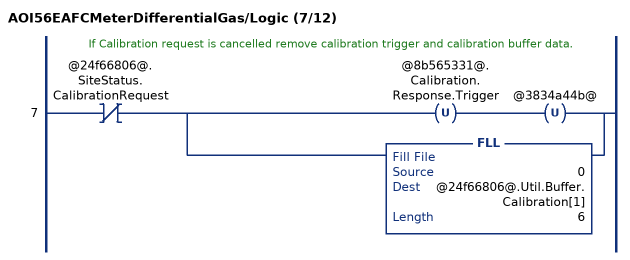
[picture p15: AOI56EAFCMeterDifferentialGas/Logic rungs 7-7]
   // If Calibration request is cancelled remove calibration trigger and calibration buffer data.
   7: XIO(@24f66806@.SiteStatus.CalibrationRequest)[OTU(@8b565331@.Calibration.Response.Trigger) OTU(@3834a44b@) ,FLL(0,@24f66806@.Util.Buffer.Calibration[1],6) ];
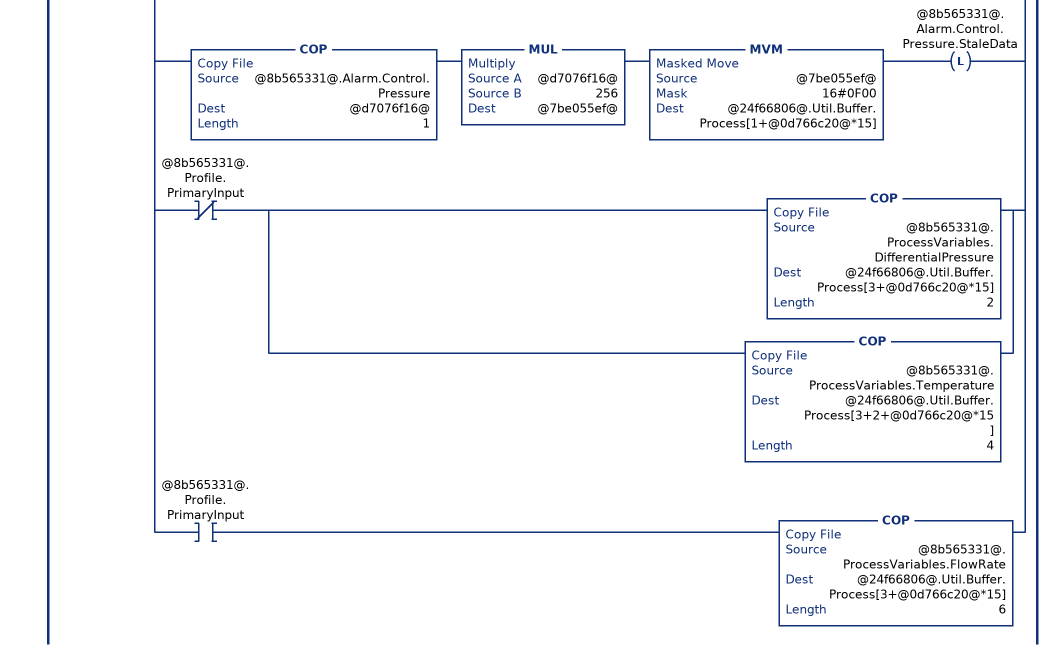
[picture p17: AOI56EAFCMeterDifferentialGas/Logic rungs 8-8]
   // Process variables and process alarms to send to module.
   8: XIC(@b5829e8f@)[ADD(16#A000,@7f34e890@,@0ce2f65c@) COP(@0ce2f65c@,@24f66806@.Util.Buffer.Process[@0d766c20@*15],1) ,[XIO(@8b565331@.Profile.PrimaryInput) XIC(@8b565331@.Alarm.Control.DifferentialPressure.SetAutoClearStaleData) OTU(@8b565331@.Alarm.Control.DifferentialPressure.StaleData) ,XIC(@8b565331@.Profile.PrimaryInput) XIC(@8b565331@.Alarm.Control.FlowRate.SetAutoClearStaleData) OTU(@8b565331@.Alarm.Control.FlowRate.StaleData) ,[XIO(@8b565331@.Profile.PrimaryInput) COP(@8b565331@.Alarm.Control.DifferentialPressure,@24f66806@.Util.Buffer.Process[1+@0d766c20@*15],1) OTL(@8b565331@.Alarm.Control.DifferentialPressure.StaleData) ,XIC(@8b565331@.Profile.PrimaryInput) COP(@8b565331@.Alarm.Control.FlowRate,@24f66806@.Util.Buffer.Process[1+@0d766c20@*15],1) OTL(@8b565331@.Alarm.Control.FlowRate.StaleData) ] ] ,[XIC(@8b565331@.Alarm.Control.Temperature.SetAutoClearStaleData) OTU(@8b565331@.Alarm.Control.Temperature.StaleData) ,COP(@8b565331@.Alarm.Control.Temperature,@d7076f16@,1) MUL(@d7076f16@,16,@7be055ef@) MVM(@7be055ef@,16#00F0,@24f66806@.Util.Buffer.Process[1+@0d766c20@*15]) OTL(@8b565331@.Alarm.Control.Temperature.StaleData) ] ,[XIC(@8b565331@.Alarm.Control.Pressure.SetAutoClearStaleData) OTU(@8b565331@.Alarm.Control.Pressure.StaleData) ,COP(@8b565331@.Alarm.Control.Pressure,@d7076f16@,1) MUL(@d7076f16@,256,@7be055ef@) MVM(@7be055ef@,16#0F00,@24f66806@.Util.Buffer.Process[1+@0d766c20@*15]) OTL(@8b565331@.Alarm.Control.Pressure.StaleData) ] ,XIO(@8b565331@.Profile.PrimaryInput) [COP(@8b565331@.ProcessVariables.DifferentialPressure,@24f66806@.Util.Buffer.Process[3+@0d766c20@*15],2) ,COP(@8b565331@.ProcessVariables.Temperature,@24f66806@.Util.Buffer.Process[3+2+@0d766c20@*15],4) ] ,XIC(@8b565331@.Profile.PrimaryInput) COP(@8b565331@.ProcessVariables.FlowRate,@24f66806@.Util.Buffer.Process[3+@0d766c20@*15],6) ];
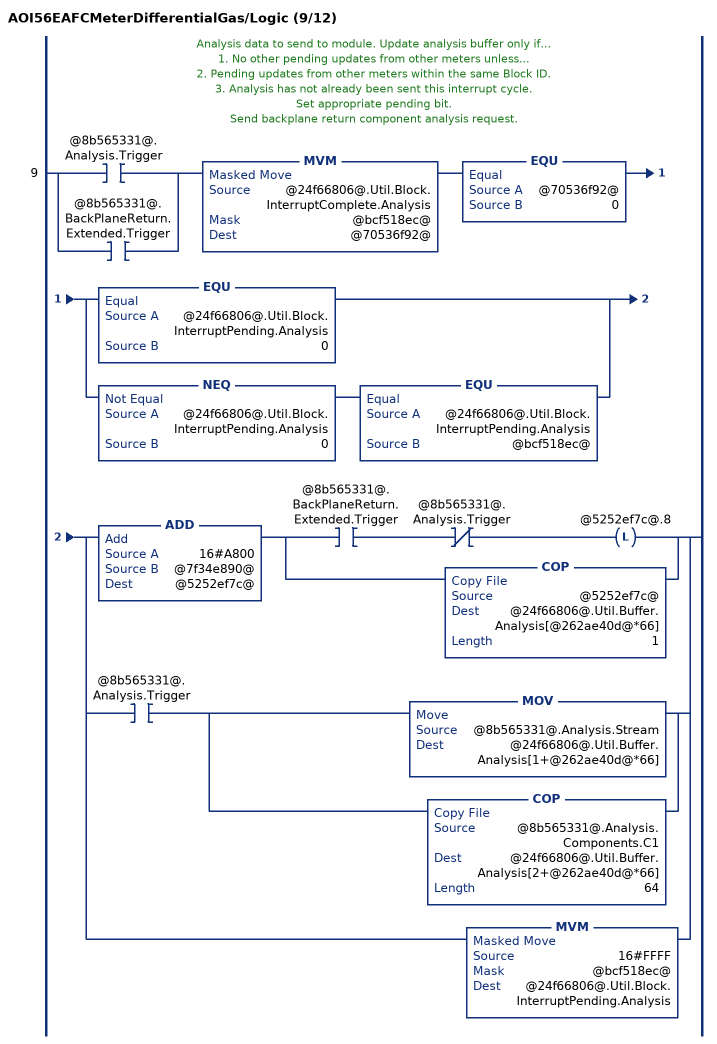
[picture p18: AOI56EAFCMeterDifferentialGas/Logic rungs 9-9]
   // Analysis data to send to module. Update analysis buffer only if...
   // 1. No other pending updates from other meters unless...
   // 2. Pending updates from other meters within the same Block ID.
   // 3. Analysis has not already been sent this interrupt cycle.
   // Set appropriate pending bit.
   // Send backplane return component analysis request.
   9: [XIC(@8b565331@.Analysis.Trigger) ,XIC(@8b565331@.BackPlaneReturn.Extended.Trigger) ]MVM(@24f66806@.Util.Block.InterruptComplete.Analysis,@bcf518ec@,@70536f92@)EQU(@70536f92@,0)[EQU(@24f66806@.Util.Block.InterruptPending.Analysis,0) ,NEQ(@24f66806@.Util.Block.InterruptPending.Analysis,0) EQU(@24f66806@.Util.Block.InterruptPending.Analysis,@bcf518ec@) ][ADD(16#A800,@7f34e890@,@5252ef7c@) [XIC(@8b565331@.BackPlaneReturn.Extended.Trigger) XIO(@8b565331@.Analysis.Trigger) OTL(@5252ef7c@.8) ,COP(@5252ef7c@,@24f66806@.Util.Buffer.Analysis[@262ae40d@*66],1) ] ,XIC(@8b565331@.Analysis.Trigger) [MOV(@8b565331@.Analysis.Stream,@24f66806@.Util.Buffer.Analysis[1+@262ae40d@*66]) ,COP(@8b565331@.Analysis.Components.C1,@24f66806@.Util.Buffer.Analysis[2+@262ae40d@*66],64) ] ,MVM(16#FFFF,@bcf518ec@,@24f66806@.Util.Block.InterruptPending.Analysis) ];
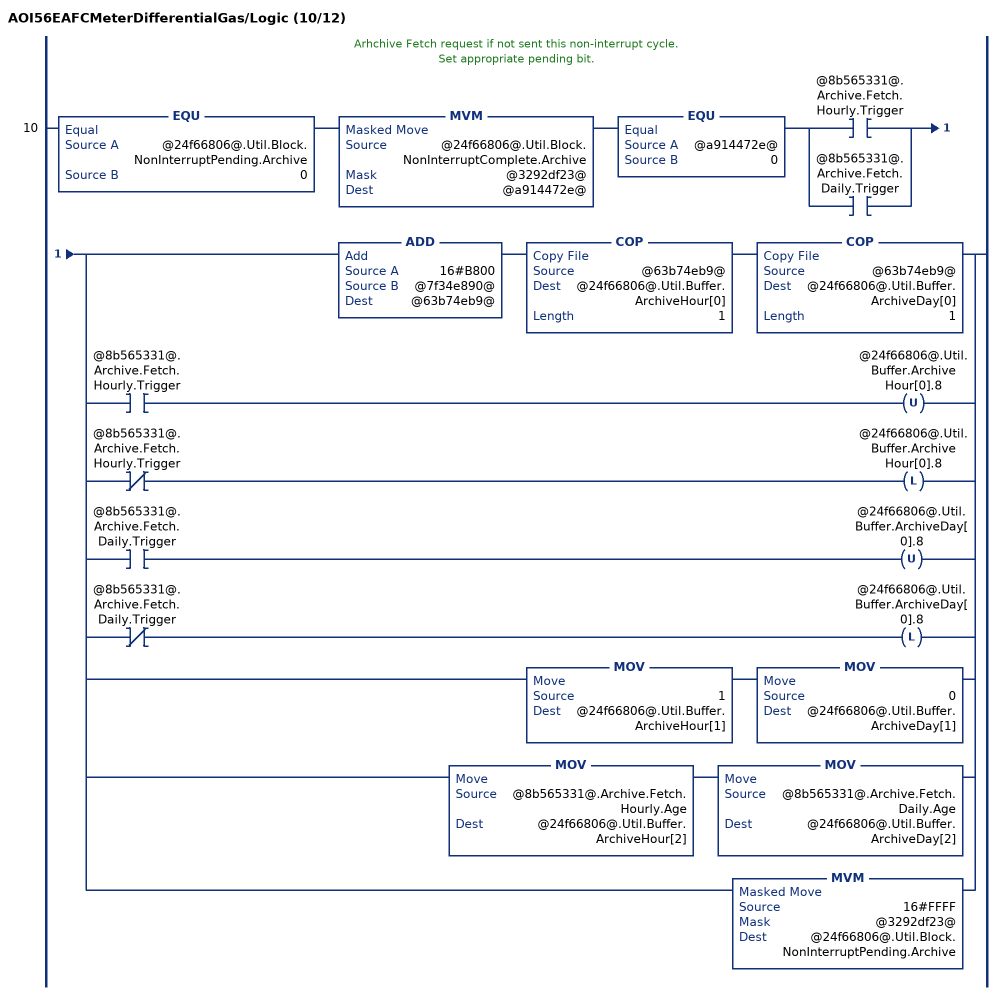
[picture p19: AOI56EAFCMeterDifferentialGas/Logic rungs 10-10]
   // Arhchive Fetch request if not sent this non-interrupt cycle.
   // Set appropriate pending bit.
   10: EQU(@24f66806@.Util.Block.NonInterruptPending.Archive,0)MVM(@24f66806@.Util.Block.NonInterruptComplete.Archive,@3292df23@,@a914472e@)EQU(@a914472e@,0)[XIC(@8b565331@.Archive.Fetch.Hourly.Trigger) ,XIC(@8b565331@.Archive.Fetch.Daily.Trigger) ][ADD(16#B800,@7f34e890@,@63b74eb9@) COP(@63b74eb9@,@24f66806@.Util.Buffer.ArchiveHour[0],1) COP(@63b74eb9@,@24f66806@.Util.Buffer.ArchiveDay[0],1) ,[XIC(@8b565331@.Archive.Fetch.Hourly.Trigger) OTU(@24f66806@.Util.Buffer.ArchiveHour[0].8) ,XIO(@8b565331@.Archive.Fetch.Hourly.Trigger) OTL(@24f66806@.Util.Buffer.ArchiveHour[0].8) ] ,[XIC(@8b565331@.Archive.Fetch.Daily.Trigger) OTU(@24f66806@.Util.Buffer.ArchiveDay[0].8) ,XIO(@8b565331@.Archive.Fetch.Daily.Trigger) OTL(@24f66806@.Util.Buffer.ArchiveDay[0].8) ] ,MOV(1,@24f66806@.Util.Buffer.ArchiveHour[1]) MOV(0,@24f66806@.Util.Buffer.ArchiveDay[1]) ,MOV(@8b565331@.Archive.Fetch.Hourly.Age,@24f66806@.Util.Buffer.ArchiveHour[2]) MOV(@8b565331@.Archive.Fetch.Daily.Age,@24f66806@.Util.Buffer.ArchiveDay[2]) ,MVM(16#FFFF,@3292df23@,@24f66806@.Util.Block.NonInterruptPending.Archive) ];
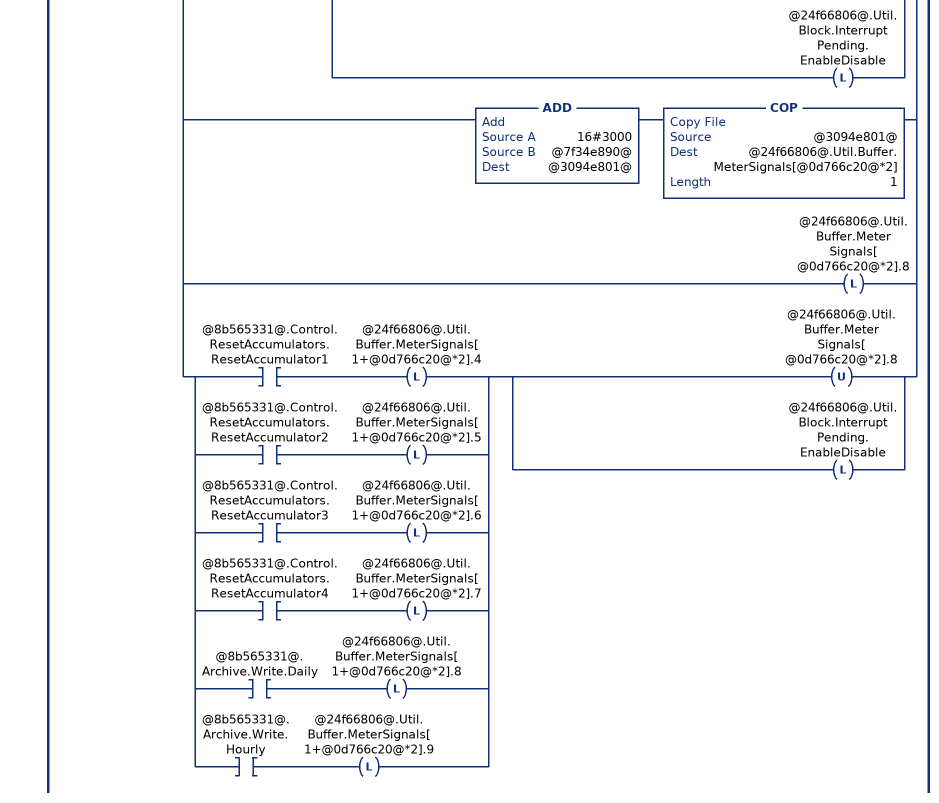
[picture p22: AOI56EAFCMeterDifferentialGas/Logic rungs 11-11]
   // Meter Enable.
   // Meter Disable.
   // Stream Select.
   // Stream Enable.
   // Stream Disable.
   // Set pending bit if not set this interrupt cycle.
   11: XIO(@24f66806@.Util.Block.InterruptComplete.EnableDisable)[LIM(1,@8b565331@.Control.Stream.Selected,16) CPT(@fec082fb@,2**(@8b565331@.Control.Stream.Selected-1)) ,[XIC(@8b565331@.Control.Meter.Enable) MVM(16#FFFF,@3292df23@,@24f66806@.Util.Buffer.MeterEnableDisable[1]) MVM(16#0000,@3292df23@,@24f66806@.Util.Buffer.MeterEnableDisable[3]) ,XIC(@8b565331@.Control.Meter.Disable) MVM(16#FFFF,@3292df23@,@24f66806@.Util.Buffer.MeterEnableDisable[3]) MVM(16#0000,@3292df23@,@24f66806@.Util.Buffer.MeterEnableDisable[1]) ] OTL(@24f66806@.Util.Block.InterruptPending.EnableDisable) ,[ADD(16#CC00,@7f34e890@,@93e49bd8@) COP(@93e49bd8@,@24f66806@.Util.Buffer.StreamEnable[@0d766c20@*3],1) ,XIO(@8b565331@.Control.Stream.EnableSelected) OTL(@24f66806@.Util.Buffer.StreamEnable[@0d766c20@*3].8) ,XIC(@8b565331@.Control.Stream.EnableSelected) [OTU(@24f66806@.Util.Buffer.StreamEnable[@0d766c20@*3].8) ,COP(@fec082fb@,@24f66806@.Util.Buffer.StreamEnable[1+@0d766c20@*3],1) ,OTL(@24f66806@.Util.Block.InterruptPending.EnableDisable) ] ] ,[ADD(16#C800,@7f34e890@,@5237ff72@) COP(@5237ff72@,@24f66806@.Util.Buffer.StreamDisable[@0d766c20@*3],1) ,XIO(@8b565331@.Control.Stream.DisableSelected) OTL(@24f66806@.Util.Buffer.StreamDisable[@0d766c20@*3].8) ,XIC(@8b565331@.Control.Stream.DisableSelected) [OTU(@24f66806@.Util.Buffer.StreamDisable[@0d766c20@*3].8) ,COP(@fec082fb@,@24f66806@.Util.Buffer.StreamDisable[1+@0d766c20@*3],1) ,OTL(@24f66806@.Util.Block.InterruptPending.EnableDisable) ] ] ,[ADD(16#3C00,@7f34e890@,@9bca9247@) COP(@9bca9247@,@24f66806@.Util.Buffer.StreamSelect[@0d766c20@*2],1) ,XIO(@8b565331@.Control.Stream.SetSelectedToActive) OTL(@24f66806@.Util.Buffer.StreamSelect[@0d766c20@*2].8) ,XIC(@8b565331@.Control.Stream.SetSelectedToActive) [OTU(@24f66806@.Util.Buffer.StreamSelect[@0d766c20@*2].8) ,MOV(@8b565331@.Control.Stream.Selected,@24f66806@.Util.Buffer.StreamSelect[1+@0d766c20@*2]) ,OTL(@24f66806@.Util.Block.InterruptPending.EnableDisable) ] ] ,[ADD(16#3000,@7f34e890@,@3094e801@) COP(@3094e801@,@24f66806@.Util.Buffer.MeterSignals[@0d766c20@*2],1) ,OTL(@24f66806@.Util.Buffer.MeterSignals[@0d766c20@*2].8) ,[XIC(@8b565331@.Control.ResetAccumulators.ResetAccumulator1) OTL(@24f66806@.Util.Buffer.MeterSignals[1+@0d766c20@*2].4) ,XIC(@8b565331@.Control.ResetAccumulators.ResetAccumulator2) OTL(@24f66806@.Util.Buffer.MeterSignals[1+@0d766c20@*2].5) ,XIC(@8b565331@.Control.ResetAccumulators.ResetAccumulator3) OTL(@24f66806@.Util.Buffer.MeterSignals[1+@0d766c20@*2].6) ,XIC(@8b565331@.Control.ResetAccumulators.ResetAccumulator4) OTL(@24f66806@.Util.Buffer.MeterSignals[1+@0d766c20@*2].7) ,XIC(@8b565331@.Archive.Write.Daily) OTL(@24f66806@.Util.Buffer.MeterSignals[1+@0d766c20@*2].8) ,XIC(@8b565331@.Archive.Write.Hourly) OTL(@24f66806@.Util.Buffer.MeterSignals[1+@0d766c20@*2].9) ] [OTU(@24f66806@.Util.Buffer.MeterSignals[@0d766c20@*2].8) ,OTL(@24f66806@.Util.Block.InterruptPending.EnableDisable) ] ] ];
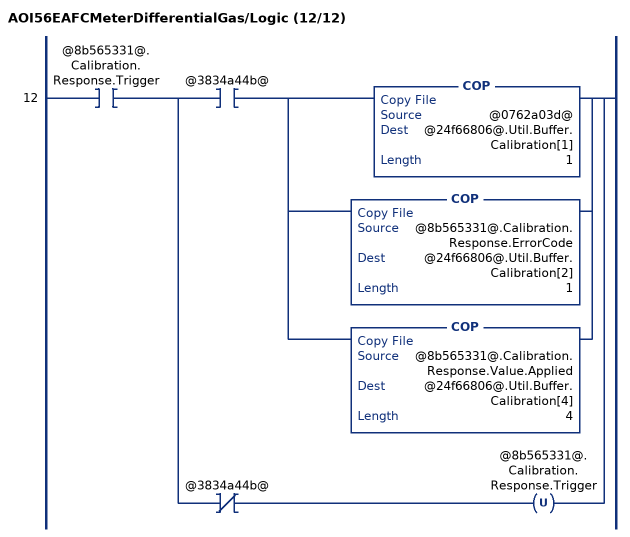
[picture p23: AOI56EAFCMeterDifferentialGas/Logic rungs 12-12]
   12: XIC(@8b565331@.Calibration.Response.Trigger)[XIC(@3834a44b@) [COP(@0762a03d@,@24f66806@.Util.Buffer.Calibration[1],1) ,COP(@8b565331@.Calibration.Response.ErrorCode,@24f66806@.Util.Buffer.Calibration[2],1) ,COP(@8b565331@.Calibration.Response.Value.Applied,@24f66806@.Util.Buffer.Calibration[4],4) ] ,XIO(@3834a44b@) OTU(@8b565331@.Calibration.Response.Trigger) ];
END_ROUTINE

ROUTINE Prescan   (* ladder *)
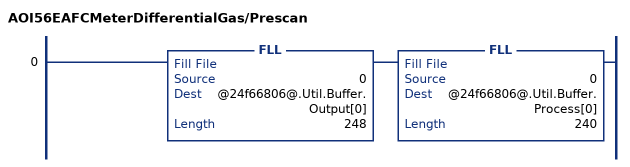
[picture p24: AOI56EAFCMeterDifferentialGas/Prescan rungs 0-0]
   0: FLL(0,@24f66806@.Util.Buffer.Output[0],248)FLL(0,@24f66806@.Util.Buffer.Process[0],240);
END_ROUTINE
END_ADD_ON_INSTRUCTION

VAR_GLOBAL   (* controller tags *)
   AFC : AFCEModuleDef;
   AOI56EAFCMeter01DifferentialGas : AOI56EAFCMeterDifferentialGas;
   AFCMeter01DifferentialGas : AFCEMeterDifferentialGas;
   Local:1:I : AB:1756_MODULE_INT_500Bytes:I:0;
END_VAR

PROGRAM MainProgram

ROUTINE MainRoutine   (* ladder *)
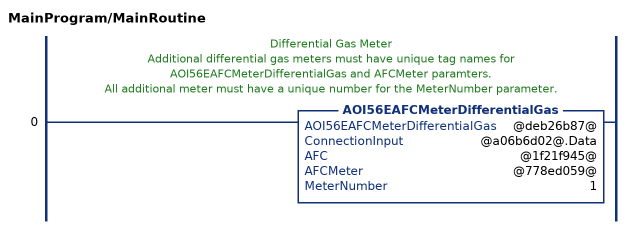
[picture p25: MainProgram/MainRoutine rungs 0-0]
   // Differential Gas Meter
   // Additional differential gas meters must have unique tag names for AOI56EAFCMeterDifferentialGas and AFCMeter paramters.
   // All additional meter must have a unique number for the MeterNumber parameter.
   0: AOI56EAFCMeterDifferentialGas(@deb26b87@,@a06b6d02@.Data,@1f21f945@,@778ed059@,1);
END_ROUTINE
END_PROGRAM
